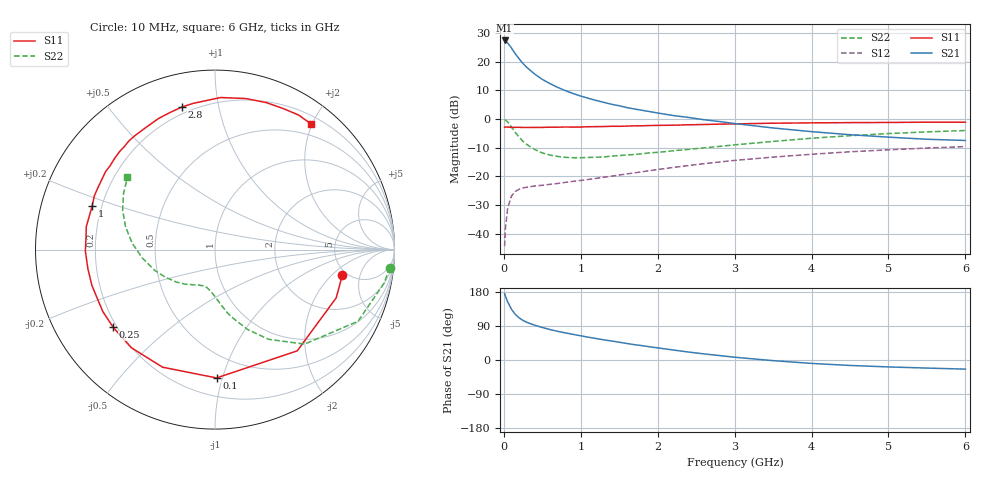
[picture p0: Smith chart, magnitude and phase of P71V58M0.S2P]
! SIEMENS Small Signal Semiconductors
! BFP196
! Si NPN RF Bipolar Junction Transistor in SOT143
! VCE = 1.5 V  IC = 8 mA
! Common Emitter S-Parameters:  May  1996
# GHz  S  MA  R  50
!  f  S11  S21  S12  S22
! GHz  MAG  ANG  MAG  ANG  MAG  ANG  MAG  ANG
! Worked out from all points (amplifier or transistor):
!   36 points, 10 MHz to 6 GHz, reference 50 ohm
!   highest |S21| = 27.4 dB at 10 MHz (marker M1)
!   |S21| within 3 dB of that: start of sweep to 108.6 MHz
!   unconditionally stable (mu >= 1): 919 MHz to 3.324 GHz
!   at 250 MHz: K = 0.35, MSG = 21.7 dB, |S12| = -24.0 dB
!   at 1.4 GHz: K = 1.16, MAG = 10.1 dB, |S12| = -19.9 dB
!   at 6 GHz: K = 1.00, MSG = 1.1 dB, |S12| = -9.6 dB
!   S11 on the Smith chart (normalised r, x): 10 MHz: 4.56, -2.72; 100 MHz: 0.33, -0.96; 250 MHz: 0.19, -0.33; 1 GHz: 0.16, +0.17; 2.8 GHz: 0.16, +0.78; 6 GHz: 0.32, +1.99
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0.01  0.7237 -11.3  23.44 175.3  0.0061 86.7  0.979 -5.9
0.02  0.7269 -21.7  22.83 168.5  0.0122 78.7  0.9607 -11.2
0.05  0.7268 -50.9  21.17 153.5  0.0283 66.4  0.8912 -26.6
0.1  0.715 -89.3  17.28 133.6  0.0459 50.0  0.7259 -46.5
0.15  0.7173 -114.0  13.64 120.1  0.055 40.6  0.5826 -59.1
0.2  0.7186 -130.5  11.19 111.0  0.06 34.9  0.4828 -67.6
0.25  0.7135 -142.6  9.264 104.2  0.0632 31.3  0.4083 -73.9
0.3  0.714 -151.1  7.911 99.3  0.065 29.6  0.3603 -78.8
0.4  0.7143 -163.7  6.102 91.9  0.0682 28.3  0.2955 -85.4
0.5  0.7163 -171.6  4.918 85.8  0.0703 28.3  0.2571 -90.8
0.6  0.7223 -179.4  4.141 80.4  0.0729 29.4  0.2357 -95.3
0.7  0.7219 174.7  3.569 75.6  0.0755 30.5  0.2233 -99.1
0.8  0.7285 169.9  3.129 71.6  0.0789 31.7  0.2154 -102.5
1  0.7264 160.3  2.519 63.8  0.0853 34.2  0.212 -108.1
1.1  0.736 155.9  2.3 60.1  0.0888 35.7  0.2144 -111.0
1.6  0.7552 138.0  1.584 43.5  0.1108 39.6  0.2366 -124.6
2.2  0.7818 119.5  1.154 26.4  0.1434 39.8  0.28 -139.5
2.8  0.8159 102.9  0.907 11.8  0.1785 36.3  0.334 -156.0
3.5  0.8478 87.9  0.7 -1.7  0.2174 29.4  0.4078 -173.4
4.5  0.8676 70.7  0.534 -14.4  0.2692 18.5  0.5139 165.7
5.5  0.8826 58.2  0.445 -21.3  0.3129 7.0  0.5983 148.4
6  0.8814 52.5  0.424 -24.1  0.3314 0.8  0.6321 140.5
